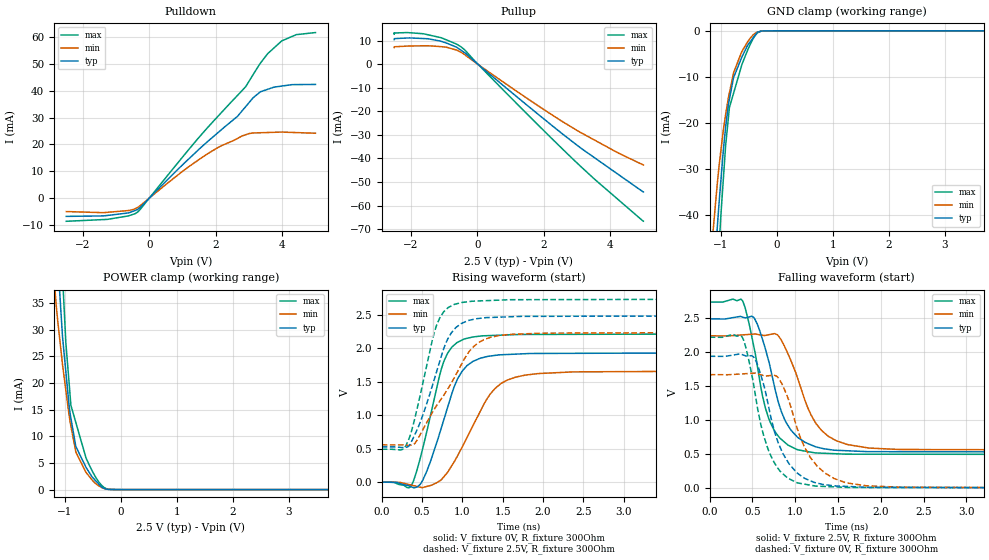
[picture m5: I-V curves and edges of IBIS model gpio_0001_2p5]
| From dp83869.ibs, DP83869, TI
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|   gpio_0001_2p5 Model
[Model]   gpio_0001_2p5
Model_type   I/O
Polarity   Non-Inverting
Enable   Active-Low
Vinl = 0.7
Vinh = 1.7
Vmeas = 1.25
Vref = 0
Cref = 2pF
Rref = 100000
|   typ   min   max
C_comp   1.246pF   1.092pF   1.323pF
| Where Nom  PVT is Nominal Process, 2.5V,  27C
|   Fast PVT is Strong Process,  2.75V, -40C
|   Slow PVT is Weak Process,   2.25V, 125C
[Voltage Range]   2.5   2.25   2.75
|Junction Temperature
[Temperature Range]   27   125   -40
[Pullup Reference]   2.5   2.25   2.75
[Pulldown Reference]   0   0   0
[Power Clamp Reference]   2.5   2.25   2.75
[GND Clamp Reference]   0   0   0
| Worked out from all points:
|   slope of the pulldown table from 0 to 0.375 V, typ, clamps not added: 79.8 ohm
|   slope of the pullup table from 0 to 0.375 V, typ, clamps not added: 84.2 ohm
|   GND clamp passes 1 mA (typ) near -0.39 V on its own axis
|   POWER clamp passes 1 mA (typ) near -0.39 V on its own axis
|   falling waveform, V_fixture 2.5V, R_fixture 300Ohm: 20-80 % time 275ps typ, 337ps min, 235ps max; typ from 2.48 V to 0.526 V
|   rising waveform, V_fixture 0V, R_fixture 300Ohm: 20-80 % time 317ps typ, 443ps min, 266ps max; typ from 0 V to 1.93 V
|   rising waveform, V_fixture 2.5V, R_fixture 300Ohm: 20-80 % time 317ps typ, 497ps min, 257ps max; typ from 0.526 V to 2.48 V
|   falling waveform, V_fixture 0V, R_fixture 300Ohm: 20-80 % time 287ps typ, 336ps min, 251ps max; typ from 1.93 V to 0 V
[Pulldown]
|   Voltage   I(typ)   I(min)   I(max)
-2.5V     -6.818mA   -5.022mA   -8.652mA
-1.268V   -6.48mA    -5.309mA   -7.941mA
-348.8mV  -4.254mA   -3.457mA   -5.17mA
976.8mV   12.12mA    9.749mA    14.93mA
1.859V    22.19mA    17.31mA    27.7mA
2.656V    30.49mA    22.24mA    38.28mA
2.904V    34.15mA    23.62mA    41.57mA
3.343V    39.61mA    24.34mA    50.25mA
3.559V    40.52mA    24.43mA    53.76mA
3.985V    41.73mA    24.59mA    58.56mA
4.422V    42.28mA    24.4mA     60.88mA
5V        42.34mA    24.15mA    61.66mA
[GND Clamp]
|   Voltage   I(typ)   I(min)   I(max)
-2.5V     -325.5mA   -278mA     -374.2mA
-1.151V   -58.23mA   -45.14mA   -72.47mA
-1.062V   -42.41mA   -32.96mA   -53.36mA
-1.027V   -36.66mA   -28.83mA   -45.98mA
-1.002V   -32.86mA   -26.25mA   -40.53mA
-914.3mV  -20.84mA   -18.12mA   -24.89mA
-846.8mV  -14.83mA   -13.46mA   -16.65mA
-770.2mV  -10.08mA   -9.023mA   -13.45mA
-624.7mV  -5.69mA    -4.486mA   -7.367mA
-460.5mV  -2.142mA   -1.389mA   -2.573mA
-358.7mV  -493.6uA   -330.5uA   -623.1uA
5V        0A         0A         0A
[Pullup]
|   Voltage   I(typ)   I(min)   I(max)
-2.5V     10.52mA    7.148mA    12.86mA
-2.499V   10.91mA    7.471mA    13.32mA
-2.497V   10.91mA    7.473mA    12.96mA
-2.496V   10.92mA    7.474mA    13.32mA
-2.109V   11.18mA    7.749mA    13.5mA
-1.473V   10.85mA    7.891mA    12.53mA
-932.2mV  9.097mA    7.277mA    10.42mA
-487.5mV  5.977mA    5.09mA     7.444mA
1.265V    -14.64mA   -12.2mA    -17.76mA
2.56V     -29.5mA    -24.29mA   -35.89mA
3.539V    -39.78mA   -32.25mA   -48.9mA
5V        -54.26mA   -42.76mA   -66.69mA
[POWER Clamp]
|   Voltage   I(typ)   I(min)   I(max)
-2.5V     383.1mA    300.3mA    465.8mA
-1.265V   71.44mA    49.26mA    97.28mA
-1.162V   48.95mA    35.07mA    69.59mA
-1.083V   35.05mA    27.13mA    48.54mA
-1.045V   28.71mA    23.46mA    40.27mA
-931.5mV  16.22mA    14.27mA    20.59mA
-894.8mV  13.41mA    11.9mA     15.81mA
-802.5mV  7.998mA    6.976mA    12.43mA
-624mV    4.16mA     3.224mA    5.913mA
-448.5mV  1.623mA    1.115mA    2.26mA
-321.9mV  342.6uA    265.3uA    575.4uA
5V        0A         0A         0A
[Ramp]
R_load = 300
|   typ   min   max
dV/dt_r   1.15862/3.15861e-10   0.995971/4.42394e-10   1.32717/2.65377e-10
dV/dt_f   1.17331/2.72905e-10   1.00636/3.33838e-10   1.34351/2.33697e-10
[Falling Waveform]
V_fixture = 2.5V
V_fixture_min = 2.25V
V_fixture_max = 2.75V
R_fixture = 300Ohm
C_fixture = 0F
|   Time   V(typ)   V(min)   V(max)
0s        2.482V     2.233V     2.729V
366.6ps   2.515V     2.245V     2.772V
521.6ps   2.493V     2.259V     2.041V
617.1ps   2.182V     2.241V     1.353V
718.9ps   1.706V     2.257V     932mV
837.7ps   1.12V      2.169V     712.1mV
1.015ns   759mV      1.659V     565.9mV
1.243ns   601.3mV    942.8mV    513.1mV
1.619ns   544.5mV    633.9mV    495.3mV
5ns       526.1mV    555.9mV    490.3mV
[Rising Waveform]
V_fixture = 0V
V_fixture_min = 0V
V_fixture_max = 0V
R_fixture = 300Ohm
C_fixture = 0F
|   Time   V(typ)   V(min)   V(max)
0s        231.1uV    391.3uV    230.5uV
370.6ps   -72.05mV   -45.07mV   -45.5mV
511.2ps   34.34mV    -80.09mV   515.6mV
766ps     914mV      73.35mV    1.785V
904.2ps   1.438V     313.9mV    2.05V
1.015ns   1.679V     562.8mV    2.13V
1.349ns   1.881V     1.318V     2.186V
1.665ns   1.909V     1.567V     2.201V
2.375ns   1.921V     1.644V     2.204V
5ns       1.931V     1.66V      2.212V
[Rising Waveform]
V_fixture = 2.5V
V_fixture_min = 2.25V
V_fixture_max = 2.75V
R_fixture = 300Ohm
C_fixture = 0F
|   Time   V(typ)   V(min)   V(max)
0s        526.1mV    556mV      490.3mV
297ps     516.8mV    552mV      537.1mV
373.8ps   616.7mV    554mV      778.3mV
475.5ps   887.3mV    705.8mV    1.287V
674.5ps   1.622V     1.129V     2.318V
783.4ps   2.038V     1.322V     2.557V
896.2ps   2.273V     1.549V     2.649V
1.139ns   2.428V     2.021V     2.699V
1.453ns   2.46V      2.185V     2.714V
5ns       2.482V     2.233V     2.729V
[Falling Waveform]
|Gnd
V_fixture = 0V
V_fixture_min = 0V
V_fixture_max = 0V
R_fixture = 300Ohm
C_fixture = 0F
|   Time   V(typ)   V(min)   V(max)
0s        1.933V     1.663V     2.213V
380.5ps   1.958V     1.674V     2.215V
515.2ps   1.921V     1.684V     1.509V
600.7ps   1.643V     1.66V      914.5mV
715.1ps   1.035V     1.651V     470.4mV
842.2ps   540.8mV    1.533V     222.2mV
1.015ns   226.3mV    900.7mV    78.85mV
1.256ns   69.88mV    318.6mV    25.07mV
1.601ns   21.61mV    72.95mV    7.158mV
5ns       227.3uV    385.1uV    229.3uV
